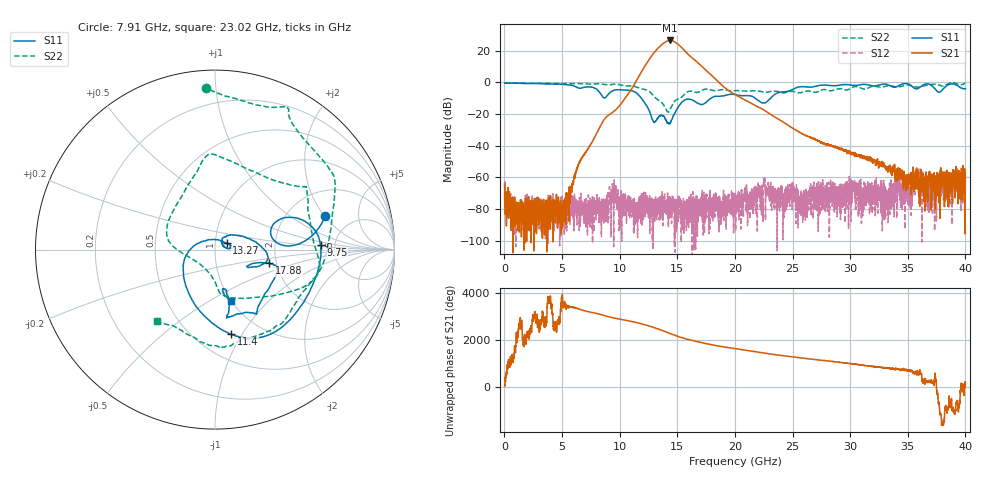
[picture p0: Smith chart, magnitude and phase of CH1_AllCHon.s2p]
!Keysight Technologies,N5245B,MY57181321,A.14.80.03
!Date: Thursday, August 24, 2023 17:13:02
!Correction: S11(C  2-Port  )
!S21(C  2-Port  )
!S12(C  2-Port  )
!S22(C  2-Port  )
!S2P File: Measurements: S11, S21, S12, S22:
# Hz S  RI  R 50
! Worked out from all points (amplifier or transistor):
!   4000 points, 10 MHz to 40 GHz, reference 50 ohm
!   highest |S21| = 26.5 dB at 14.36 GHz (marker M1)
!   |S21| within 3 dB of that: 13.59 GHz to 15.16 GHz (1.571 GHz wide, 10.9 % of centre)
!   unconditionally stable (mu >= 1): start of sweep to end of sweep
!   at 6.67 GHz: K = 139771.89, MAG = -37.4 dB, |S12| = -81.9 dB
!   at 20.01 GHz: K = 9705.75, MAG = -5.3 dB, |S12| = -82.8 dB
!   at 40 GHz: K = 31895.18, MAG = -44.6 dB, |S12| = -66.3 dB
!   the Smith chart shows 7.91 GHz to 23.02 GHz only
!   S11 on the Smith chart (normalised r, x): 7.91 GHz: 3.18, +2.06; 9.75 GHz: 3.84, +0.28; 11.4 GHz: 0.73, -0.90; 13.27 GHz: 1.14, +0.08; 17.88 GHz: 1.83, -0.31; 23.02 GHz: 1.00, -0.62
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1e7  -0.9569 0.0445  0.000311 0.000539  -0.000716 0.000146  -0.9613 0.0213
6.68e9  0.3519 0.5646  0.00338 0.00214  8.51e-06 0.000181  -0.3462 0.847
7.91e9  0.6146 0.1897  -0.00632 -0.0203  0.000163 -7.74e-05  -0.0513 0.9028
9.75e9  0.5878 0.0241  0.132 0.0673  -1.54e-05 -9.27e-05  0.4105 0.7782
1.14e10  0.0897 -0.4719  -0.6989 -0.7816  1.74e-05 4.62e-05  0.6656 0.3042
1.267e10  -0.0951 0.0344  3.431 5.074  -6.67e-05 -6.92e-05  0.4201 -0.2345
1.327e10  0.0647 0.0357  8.646 -7.743  -0.000174 -6.82e-05  0.1091 -0.2704
1.334e10  0.0702 0.0307  7.303 -9.912  -0.000117 0.000166  0.0837 -0.2677
1.368e10  0.0897 0.00799  -6.182 -14.85  0.000268 0.000227  0.02 -0.2269
1.399e10  0.0649 0.00931  -18.97 -3.611  0.000157 8.95e-05  -0.02 -0.1469
1.436e10  0.0396 0.0299  -10.83 18.27  -2.15e-05 -7.2e-05  -0.1269 -0.0519
1.461e10  0.0466 0.0665  5.755 19.53  -1.93e-05 -0.00016  -0.2121 -0.000372
1.495e10  0.1156 0.0808  16.8 3.955  -0.00015 -3.22e-05  -0.2692 0.0929
1.541e10  0.2368 0.0341  6.09 -10.7  -3.88e-05 -8.34e-05  -0.1849 0.2986
1.604e10  0.2922 -0.0577  -5.804 -4.162  1.33e-05 -5.57e-05  -0.0388 0.5283
1.68e10  0.1937 -0.0989  -2.452 3.358  1.56e-06 4.9e-05  0.2672 0.4113
1.788e10  0.3018 -0.0754  1.756 0.3777  -3.48e-05 8.43e-05  0.5191 0.2679
2.001e10  0.2159 -0.3547  -0.3873 -0.1412  6.9e-05 -2.17e-05  0.4048 -0.3692
2.302e10  0.0876 -0.2853  0.0929 -0.0412  0.000172 -4.7e-05  -0.3207 -0.3985
2.667e10  -0.1202 -0.7074  -0.00757 0.0164  -8.04e-05 0.000163  -0.3259 0.3959
3.334e10  -0.823 0.0347  9.53e-05 0.00173  0.000154 -0.000102  0.7654 -0.1853
4e10  0.3104 0.5567  -0.000633 0.000862  -0.000365 0.000321  0.2099 -0.9487
